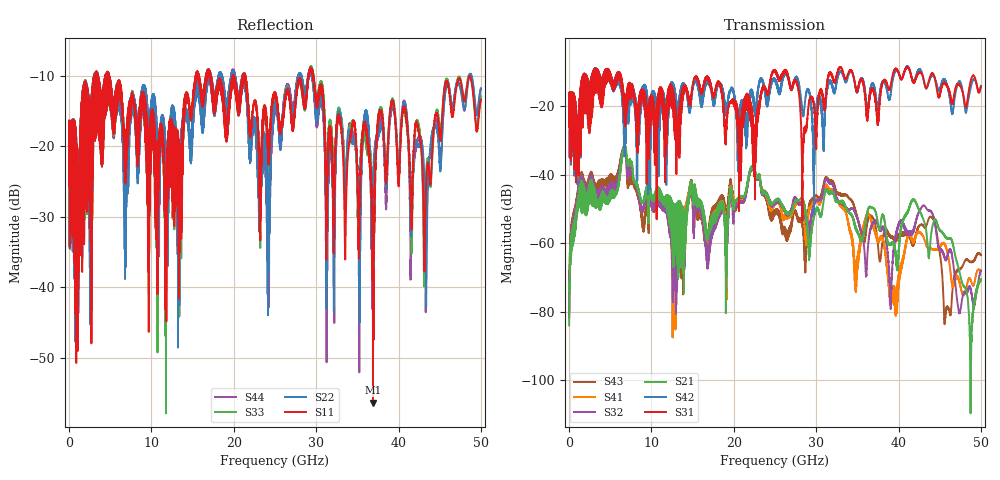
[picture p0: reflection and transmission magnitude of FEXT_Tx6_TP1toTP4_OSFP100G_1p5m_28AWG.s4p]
! Touchstone data
! Created: 27-Feb-2019 by IdEM 12 (12.1.0)
! COMMENTS
!  Created Wed Feb 27 09:43:39 2019
!  64 Port Network Data from SP1.SP block
!  freq  magS1_1  angS1_1  magS1_2  angS1_2  magS1_3  angS1_3  magS1_4  angS1_4
!  magS1_5  angS1_5  magS1_6  angS1_6  magS1_7  angS1_7  magS1_8  angS1_8
!  magS1_9  angS1_9  magS1_10  angS1_10  magS1_11  angS1_11  magS1_12  angS1_12
!  magS1_13  angS1_13  magS1_14  angS1_14  magS1_15  angS1_15  magS1_16  angS1_16
!  magS1_17  angS1_17  magS1_18  angS1_18  magS1_19  angS1_19  magS1_20  angS1_20
!  magS1_21  angS1_21  magS1_22  angS1_22  magS1_23  angS1_23  magS1_24  angS1_24
!  magS1_25  angS1_25  magS1_26  angS1_26  magS1_27  angS1_27  magS1_28  angS1_28
!  magS1_29  angS1_29  magS1_30  angS1_30  magS1_31  angS1_31  magS1_32  angS1_32
!  magS1_33  angS1_33  magS1_34  angS1_34  magS1_35  angS1_35  magS1_36  angS1_36
!  magS1_37  angS1_37  magS1_38  angS1_38  magS1_39  angS1_39  magS1_40  angS1_40
!  magS1_41  angS1_41  magS1_42  angS1_42  magS1_43  angS1_43  magS1_44  angS1_44
!  magS1_45  angS1_45  magS1_46  angS1_46  magS1_47  angS1_47  magS1_48  angS1_48
!  magS1_49  angS1_49  magS1_50  angS1_50  magS1_51  angS1_51  magS1_52  angS1_52
!  magS1_53  angS1_53  magS1_54  angS1_54  magS1_55  angS1_55  magS1_56  angS1_56
!  magS1_57  angS1_57  magS1_58  angS1_58  magS1_59  angS1_59  magS1_60  angS1_60
!  magS1_61  angS1_61  magS1_62  angS1_62  magS1_63  angS1_63  magS1_64  angS1_64
!  magS2_1  angS2_1  magS2_2  angS2_2  magS2_3  angS2_3  magS2_4  angS2_4
!  magS2_5  angS2_5  magS2_6  angS2_6  magS2_7  angS2_7  magS2_8  angS2_8
!  magS2_9  angS2_9  magS2_10  angS2_10  magS2_11  angS2_11  magS2_12  angS2_12
!  magS2_13  angS2_13  magS2_14  angS2_14  magS2_15  angS2_15  magS2_16  angS2_16
!  magS2_17  angS2_17  magS2_18  angS2_18  magS2_19  angS2_19  magS2_20  angS2_20
!  magS2_21  angS2_21  magS2_22  angS2_22  magS2_23  angS2_23  magS2_24  angS2_24
!  magS2_25  angS2_25  magS2_26  angS2_26  magS2_27  angS2_27  magS2_28  angS2_28
!  magS2_29  angS2_29  magS2_30  angS2_30  magS2_31  angS2_31  magS2_32  angS2_32
!  magS2_33  angS2_33  magS2_34  angS2_34  magS2_35  angS2_35  magS2_36  angS2_36
!  magS2_37  angS2_37  magS2_38  angS2_38  magS2_39  angS2_39  magS2_40  angS2_40
!  magS2_41  angS2_41  magS2_42  angS2_42  magS2_43  angS2_43  magS2_44  angS2_44
!  magS2_45  angS2_45  magS2_46  angS2_46  magS2_47  angS2_47  magS2_48  angS2_48
!  magS2_49  angS2_49  magS2_50  angS2_50  magS2_51  angS2_51  magS2_52  angS2_52
!  magS2_53  angS2_53  magS2_54  angS2_54  magS2_55  angS2_55  magS2_56  angS2_56
!  magS2_57  angS2_57  magS2_58  angS2_58  magS2_59  angS2_59  magS2_60  angS2_60
!  magS2_61  angS2_61  magS2_62  angS2_62  magS2_63  angS2_63  magS2_64  angS2_64
!  magS3_1  angS3_1  magS3_2  angS3_2  magS3_3  angS3_3  magS3_4  angS3_4
!  magS3_5  angS3_5  magS3_6  angS3_6  magS3_7  angS3_7  magS3_8  angS3_8
!  magS3_9  angS3_9  magS3_10  angS3_10  magS3_11  angS3_11  magS3_12  angS3_12
!  magS3_13  angS3_13  magS3_14  angS3_14  magS3_15  angS3_15  magS3_16  angS3_16
!  magS3_17  angS3_17  magS3_18  angS3_18  magS3_19  angS3_19  magS3_20  angS3_20
!  magS3_21  angS3_21  magS3_22  angS3_22  magS3_23  angS3_23  magS3_24  angS3_24
!  magS3_25  angS3_25  magS3_26  angS3_26  magS3_27  angS3_27  magS3_28  angS3_28
!  magS3_29  angS3_29  magS3_30  angS3_30  magS3_31  angS3_31  magS3_32  angS3_32
!  magS3_33  angS3_33  magS3_34  angS3_34  magS3_35  angS3_35  magS3_36  angS3_36
!  magS3_37  angS3_37  magS3_38  angS3_38  magS3_39  angS3_39  magS3_40  angS3_40
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# Hz S MA R 50
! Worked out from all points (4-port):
!   5000 points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, 10 MHz to 50 GHz, reference 50 ohm
!   strongest paths, dB at 10 MHz, 12.51 GHz, 25.01 GHz, 37.51 GHz, 50 GHz:
!     S31: -19.6, -16.6, -9.8, -25.4, -14.2
!     S42: -19.6, -15.1, -12.3, -20.3, -14.0
!     S21: -83.9, -47.9, -47.5, -54.3, -70.6
!     S32: -81.5, -50.0, -47.9, -54.9, -67.9
!     S41: -81.7, -50.4, -48.1, -58.9, -67.9
!     S43: -79.8, -49.2, -50.2, -60.7, -63.4
!   lowest |S11| = -56.3 dB at 36.9 GHz (marker M1), VSWR 1.00, Z = 50.1 + j0.121 ohm
!   |S11| at or under -10 dB: 4.861 GHz to 15.4 GHz (10.54 GHz wide, 104 % of centre); 21.38 GHz to 29.07 GHz (7.682 GHz wide, 30.5 % of centre); 29.66 GHz to end of sweep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
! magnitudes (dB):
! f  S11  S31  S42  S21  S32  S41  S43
! 10 MHz  -19.1  -19.6  -19.6  -83.9  -81.5  -81.7  -79.8
! 1.31 GHz  -28.0  -26.0  -27.0  -43.1  -41.4  -41.5  -40.2
! 6.7 GHz  -21.9  -22.9  -32.0  -31.5  -31.6  -31.7  -32.0
! 16.85 GHz  -9.2  -12.1  -12.7  -58.6  -67.2  -60.3  -58.4
! 22.22 GHz  -15.9  -25.4  -16.9  -37.4  -38.1  -37.7  -38.0
! 36.9 GHz  -56.3  -14.9  -13.2  -49.7  -54.0  -54.7  -52.6
! 50 GHz  -13.4  -14.2  -14.0  -70.6  -67.9  -67.9  -63.4
